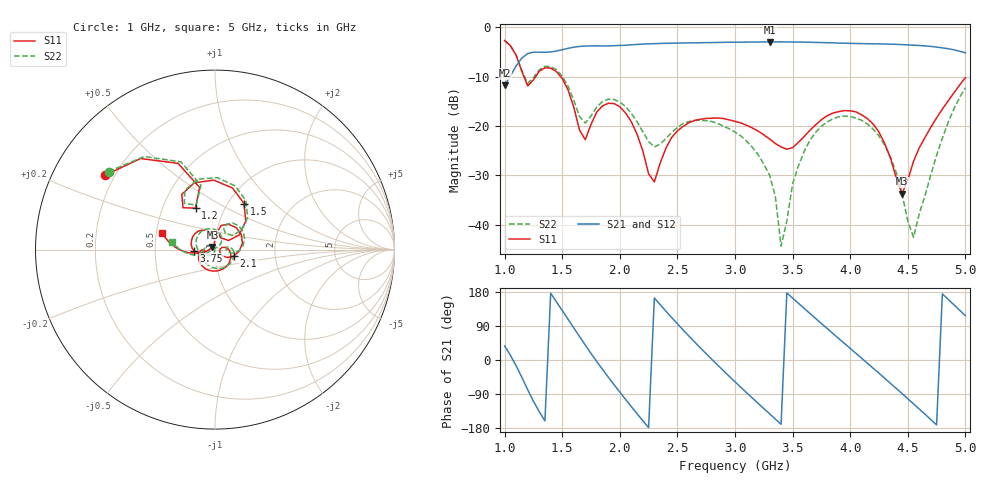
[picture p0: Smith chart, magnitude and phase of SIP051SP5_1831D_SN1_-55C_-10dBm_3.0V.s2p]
# GHz  S  dB  R  50
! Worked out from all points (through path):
!   81 points, 1 GHz to 5 GHz, reference 50 ohm
!   highest |S21| = -2.92 dB at 3.3 GHz (marker M1); lowest = -11.7 dB at 1 GHz (marker M2)
!   lowest |S11| = -33.7 dB at 4.45 GHz (marker M3), VSWR 1.04, Z = 48.6 + j1.43 ohm
!   |S11| at or under -10 dB: 1.168 GHz to 1.268 GHz (100.5 MHz wide, 8.25 % of centre); 1.487 GHz to end of sweep
!   |S22| runs from -44.4 to -2.7 dB; largest |S21 - S12| = 0.0019
!   S11 on the Smith chart (normalised r, x): 1 GHz: 0.16, +0.30; 1.2 GHz: 0.73, +0.36; 1.5 GHz: 1.18, +0.67; 2.1 GHz: 1.23, -0.09; 3.75 GHz: 0.79, -0.01; 5 GHz: 0.54, +0.11
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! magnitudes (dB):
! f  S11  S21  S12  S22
! 1 GHz  -2.6  -11.7  -11.7  -2.7
! 1.2 GHz  -11.9  -5.3  -5.3  -11.4
! 1.35 GHz  -8.2  -5.0  -5.0  -7.9
! 1.5 GHz  -10.4  -4.5  -4.5  -9.9
! 1.7 GHz  -22.8  -3.8  -3.8  -19.4
! 1.9 GHz  -15.4  -3.7  -3.7  -14.6
! 2.1 GHz  -19.1  -3.5  -3.5  -17.4
! 2.25 GHz  -29.7  -3.3  -3.3  -23.2
! 2.35 GHz  -27.5  -3.2  -3.2  -23.7
! 2.6 GHz  -19.3  -3.1  -3.1  -19.1
! 3 GHz  -19.0  -3.0  -3.0  -21.2
! 3.3 GHz  -22.6  -2.9  -2.9  -29.9
! 3.4 GHz  -24.2  -2.9  -2.9  -44.4
! 3.5 GHz  -24.4  -3.0  -3.0  -31.8
! 3.7 GHz  -19.8  -3.0  -3.0  -21.3
! 3.75 GHz  -18.7  -3.1  -3.1  -20.0
! 4.1 GHz  -17.7  -3.3  -3.3  -18.8
! 4.35 GHz  -26.5  -3.4  -3.4  -26.4
! 4.45 GHz  -33.7  -3.5  -3.5  -33.7
! 4.55 GHz  -27.1  -3.6  -3.6  -42.6
! 4.8 GHz  -16.6  -4.1  -4.1  -22.5
! 5 GHz  -10.2  -5.1  -5.1  -12.2
